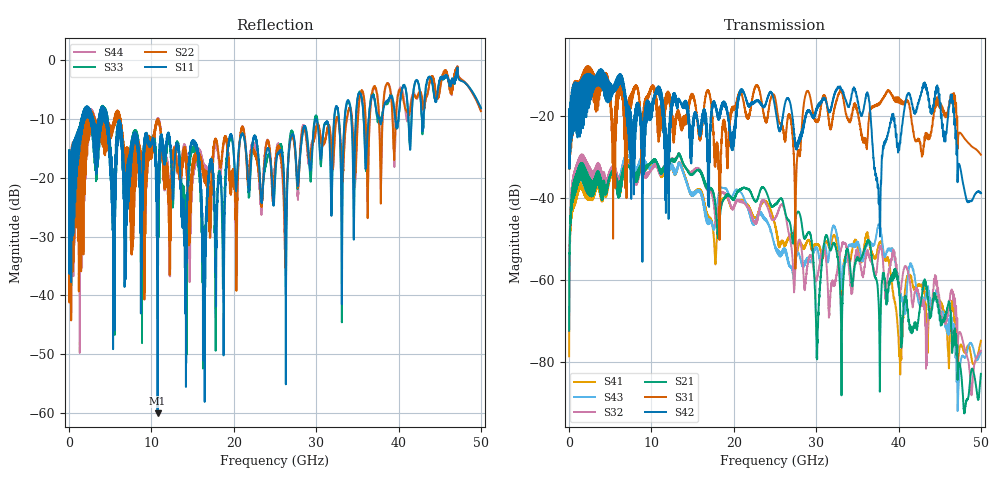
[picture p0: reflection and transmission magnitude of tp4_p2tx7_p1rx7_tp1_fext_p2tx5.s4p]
! 100G CR Analysis
! File: tp4_p2tx7_p1rx7_tp1_fext_p2tx5
! Description: 2m Cu Cable, OSFP, TP1-TP4
! Port Mapping
! Port1 -- P1RX7N
! Port2 -- P2TX5N
! Port3 -- P1RX7P
! Port4 -- P2TX5P
# GHz S MA R 50.00
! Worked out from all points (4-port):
!   5000 points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, 10 MHz to 50 GHz, reference 50 ohm
!   strongest paths, dB at 10 MHz, 12.51 GHz, 25.01 GHz, 37.51 GHz, 50 GHz:
!     S42: -20.5, -15.9, -17.8, -36.7, -38.8
!     S31: -20.6, -20.0, -15.5, -17.2, -29.4
!     S21: -72.3, -30.9, -41.5, -62.6, -82.8
!     S32: -66.5, -30.9, -44.8, -54.8, -77.2
!     S43: -72.0, -32.7, -52.0, -47.2, -77.6
!     S41: -78.6, -32.8, -46.5, -52.1, -74.7
!   lowest |S11| = -60.0 dB at 10.75 GHz (marker M1), VSWR 1.00, Z = 50.1 + j0.032 ohm
!   |S11| at or under -10 dB: start of sweep to 1.499 GHz; 4.65 GHz to 32.18 GHz (27.53 GHz wide, 149 % of centre); 32.77 GHz to 33.46 GHz (687.9 MHz wide, 2.08 % of centre)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
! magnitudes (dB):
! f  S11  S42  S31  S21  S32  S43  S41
! 10 MHz  -17.8  -20.5  -20.6  -72.3  -66.5  -72.0  -78.6
! 1.29 GHz  -12.4  -12.2  -11.5  -35.6  -33.4  -35.8  -37.8
! 10.75 GHz  -60.0  -12.9  -20.5  -31.8  -32.8  -31.7  -31.9
! 36.2 GHz  -13.2  -14.2  -26.4  -50.5  -52.8  -50.8  -48.3
! 37.65 GHz  -9.8  -41.5  -17.1  -70.0  -52.9  -46.9  -51.2
! 43.21 GHz  -6.0  -12.9  -25.9  -60.7  -70.1  -64.9  -64.2
! 50 GHz  -8.1  -38.8  -29.4  -82.8  -77.2  -77.6  -74.7
